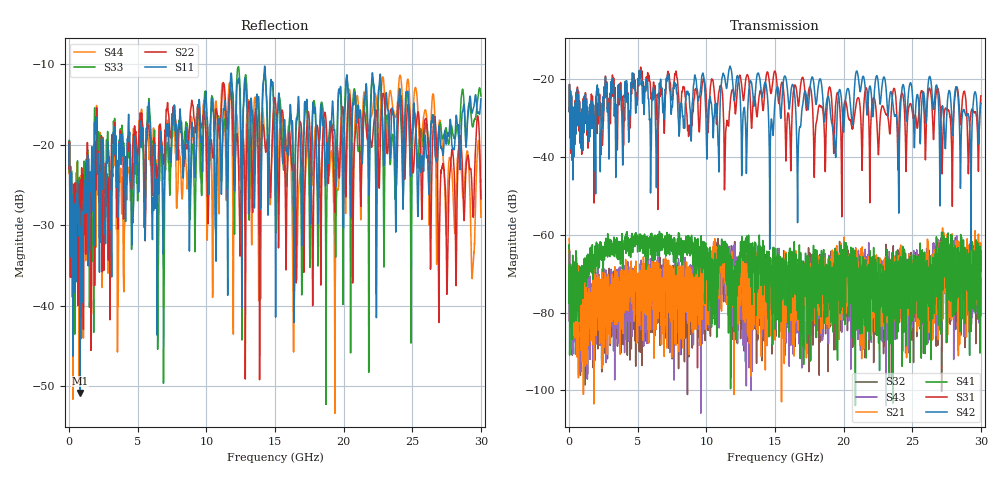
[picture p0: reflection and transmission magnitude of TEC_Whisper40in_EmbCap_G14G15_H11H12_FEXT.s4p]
! Tyco Electronics
! H11H12-G14G15_FEXT
!! PART DESCRIPTION: Whisper 40in Megtron 6 VLP-HVLP-VLP Channel, Embedded Capactior Connecter at one end, bulkhead 2.4mm test pts
!! MODEL DESCRIPTION: System 4-port S-parameter
!! MODEL STATUS: Measured
!! MODEL GEOMETRY: Channel Model
!! MODEL FREQUENCY RANGE: DC to 30.000 GHz in 10.000 MHz frequency steps
!! MODEL EDGE RATE LIMITATION: 12.500 ps (Using conservative 0.5/Fmax rule of thumb)
!! TIME-DOMAIN TRANSFORM CAUTIONS:
!! 1.) Do not simulate transient edge rates faster than the number listed above.  Edge rates faster than this number
!!  contain significant spectral content at frequencies above the model's highest frequency.
!! 2.) Even when simulating edge rates that are slower than the number listed above, be aware that the best time
!!  resolution possible with a direct iFFT is (1 / 2Fmax).  As a result, time resolution is typically not adequate
!!  for most time-domain simulations unless tricks such as windowing are used to minimize leakage and aliasing.
!! 3.) Because the model has a uniform frequency step, a direct iFFT will result in an impulse that that has a time
!!  length given by either (1 / Fstep) or (1 / 2Fstep), depending on the transform being used.  Care has been taken
!!  in selecting the frequency step to ensure a settled impulse response for the model.  Therefore, convolution with
!!  the model's impulse response should present no issues.  However, if directly concatenating s-parameter models
!!  in the frequency domain a user must either interpolate necessary interim frequencies or complete impulse response
!!  zero-padding.  Impulse response zero-padding is more difficult, but more accurate.
!! PORT DEFINITIONS:
!! Port  1  ----->  Side A  H11  G14  Side B  <-----  Port  2
!! Port  3  ----->  Side A  H12  G15  Side B  <-----  Port  4
! Point-to-Point link (differential)  !
! Connectors:  !
!  1: STRADA Whisper  !
! Materials:  !
!  Backplane: Megtron-6 HVLP  !
!  Daughtercard: Megtron-6 VLP  !
! Stack-up:  !
!  Backplane: 20 layers, 200mil thick  !
!  Daughtercard: 14 layers, 110mil thick  !
! Trace Length:  !
!  Backplane: 30in  !
!  Daightercards: 5in  !
! Trace Width:  !
!  Backplane: 7-9-7 mils  !
!  Daughtercards: 6-9-6 mils  !
! Geometry:  !
!  Backplane: Stripline  !
!  Daughtercards: Stripline  !
! Freq. Range: 0 GHz - 30 GHz  !
! Note1: non-mixed-mode s-parameters  !
! Note2: channel includes 2.4mm test points  !
! Touchstone data
! Created: 02-Jul-2013 by IdEM R2011 (7.0.3)
# Hz S MA R 50
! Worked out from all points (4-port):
!   3000 points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, 10 MHz to 30 GHz, reference 50 ohm
!   strongest paths, dB at 10 MHz, 7.51 GHz, 15.01 GHz, 22.51 GHz, 30 GHz:
!     S42: -28.3, -26.9, -25.3, -20.4, -26.1
!     S31: -28.2, -24.9, -17.9, -38.2, -24.2
!     S41: -63.4, -63.0, -73.5, -75.0, -68.8
!     S21: -61.0, -68.2, -80.0, -73.4, -68.5
!     S43: -66.3, -74.2, -76.8, -77.0, -80.8
!     S32: -69.5, -77.2, -69.8, -72.2, -66.4
!   lowest |S11| = -50.8 dB at 810 MHz (marker M1), VSWR 1.01, Z = 49.9 + j0.275 ohm
!   |S11| at or under -10 dB: start of sweep to end of sweep
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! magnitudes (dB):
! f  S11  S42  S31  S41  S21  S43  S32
! 10 MHz  -22.5  -28.3  -28.2  -63.4  -61.0  -66.3  -69.5
! 810 MHz  -50.8  -33.0  -36.4  -73.1  -78.5  -70.9  -79.7
! 11.2 GHz  -17.4  -18.8  -24.8  -62.0  -68.9  -63.6  -65.5
! 16.01 GHz  -20.9  -27.2  -29.1  -85.0  -69.4  -76.1  -78.9
! 16.45 GHz  -29.5  -24.4  -21.4  -65.9  -67.3  -74.7  -76.5
! 20.41 GHz  -15.1  -23.4  -30.3  -67.4  -66.4  -77.4  -70.7
! 30 GHz  -14.3  -26.1  -24.2  -68.8  -68.5  -80.8  -66.4
